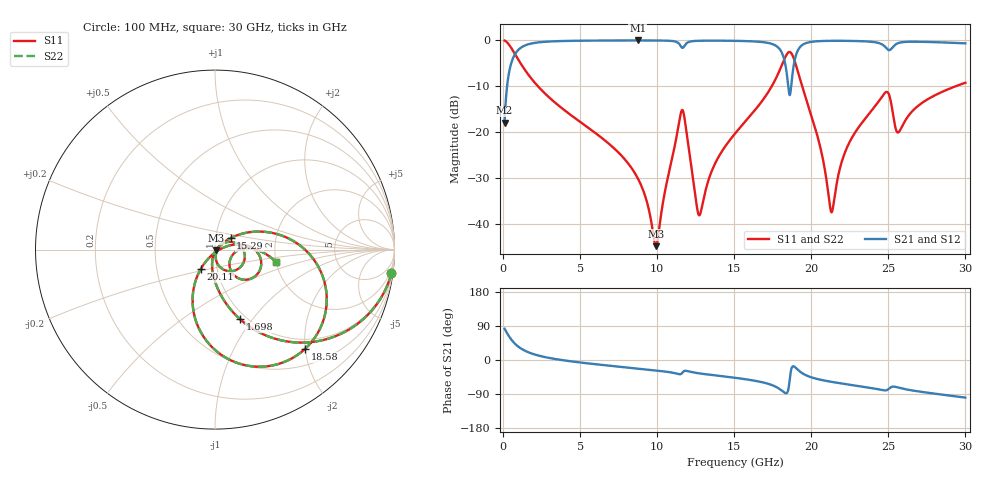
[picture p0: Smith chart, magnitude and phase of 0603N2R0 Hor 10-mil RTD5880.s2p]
# GHz S MA R 50
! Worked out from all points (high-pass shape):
!   3201 points, 100 MHz to 30 GHz, reference 50 ohm
!   highest |S21| = -0.04 dB at 8.734 GHz (marker M1); lowest = -17.9 dB at 100 MHz (marker M2)
!   |S21| within 3 dB of the highest: 771 MHz to 18.13 GHz (17.36 GHz wide, 184 % of centre); 19.03 GHz to end of sweep
!   lowest |S11| = -44.7 dB at 9.92 GHz (marker M3), VSWR 1.01, Z = 50.5 - j0.315 ohm
!   |S11| at or under -10 dB: 2.264 GHz to 17.43 GHz (15.17 GHz wide, 154 % of centre); 19.41 GHz to 29.36 GHz (9.95 GHz wide, 40.8 % of centre)
!   |S22| runs from -44.7 to -0.1 dB; largest |S21 - S12| = 0
!   S11 on the Smith chart (normalised r, x): 100 MHz: 1, -15; 1.698 GHz: 0.93, -0.87; 15.29 GHz: 1.18, +0.15; 18.58 GHz: 0.80, -1.99; 20.11 GHz: 0.84, -0.18; 30 GHz: 1.99, -0.31
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0.1  0.9918 -7.6  0.1274 82.4  0.1274 82.4  0.9918 -7.6
0.6045625  0.7889 -39.6  0.614 50.4  0.614 50.4  0.7889 -39.6
1.697781  0.4107 -70.3  0.9104 19.5  0.9104 19.5  0.4107 -70.3
5.089563  0.1267 -95.7  0.9892 -7.0  0.9892 -7.0  0.1267 -95.7
8.733625  0.03182 -104.9  0.9952 -22.5  0.9952 -22.5  0.03182 -104.9
9.920281  0.005793 -32.6  0.9941 -27.5  0.9941 -27.5  0.005793 -32.6
10.06978  0.007545 6.5  0.9936 -28.2  0.9936 -28.2  0.007545 6.5
11.58347  0.1713 -13.8  0.8388 -35.8  0.8388 -35.8  0.1713 -13.8
12.73275  0.01253 -23.4  0.9876 -35.3  0.9876 -35.3  0.01253 -23.4
13.67647  0.04286 38.2  0.9903 -40.1  0.9903 -40.1  0.04286 38.2
15.05  0.09683 37.5  0.9858 -46.9  0.9858 -46.9  0.09683 37.5
15.29294  0.1083 36.6  0.9841 -48.2  0.9841 -48.2  0.1083 36.6
17.78772  0.4114 8.9  0.8526 -72.6  0.8526 -72.6  0.4114 8.9
18.58194  0.7468 -47.9  0.2564 -58.7  0.2564 -58.7  0.7468 -47.9
19.12388  0.4607 -100.3  0.7739 -25.6  0.7739 -25.6  0.4607 -100.3
20.03956  0.1459 -125.7  0.9629 -46.1  0.9629 -46.1  0.1459 -125.7
20.11431  0.1329 -126.4  0.9664 -47.1  0.9664 -47.1  0.1329 -126.4
21.329  0.01357 -50.8  0.9862 -57.8  0.9862 -57.8  0.01357 -50.8
22.46894  0.07737 15.8  0.9843 -65.0  0.9843 -65.0  0.07737 15.8
25.01978  0.2624 -36.9  0.7837 -76.6  0.7837 -76.6  0.2624 -36.9
25.64581  0.09973 -23.1  0.9323 -72.8  0.9323 -72.8  0.09973 -23.1
30  0.3458 -11.3  0.9256 -99.2  0.9256 -99.2  0.3458 -11.3
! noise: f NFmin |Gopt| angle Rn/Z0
0.1  0.0004482  0.9484  0.9358  0.001948
3.417  0.004029  0.8097  9.846  0.004379
6.743  0.006915  0.7851  18.96  0.006437
10.06  0.0116  0.8079  27.94  0.01184
13.39  0.01614  0.8171  36.91  0.01663
16.7  0.02534  0.8534  45.59  0.03139
20.03  0.03393  0.8692  54.46  0.0442
23.35  0.02749  0.8193  62.63  0.02333
26.67  0.03325  0.8305  70.82  0.02757
30  0.02848  0.7859  78.39  0.01658
